(* Logix 5000 Rung export; software revision 16.04 *)

MODULES
   Local : vendor None type None code None
   MVI69E_AFC : vendor None type None code None
END_MODULES

TYPE AFCESiteAlarms :   // Indicates if a meter has any alarms
STRUCT
   Meter1 : BOOL;   // Meter in alarm
   Meter2 : BOOL;   // Meter in alarm
   Meter3 : BOOL;   // Meter in alarm
   Meter4 : BOOL;   // Meter in alarm
   Meter5 : BOOL;   // Meter in alarm
   Meter6 : BOOL;   // Meter in alarm
   Meter7 : BOOL;   // Meter in alarm
   Meter8 : BOOL;   // Meter in alarm
   Meter9 : BOOL;   // Meter in alarm
   Meter10 : BOOL;   // Meter in alarm
   Meter11 : BOOL;   // Meter in alarm
   Meter12 : BOOL;   // Meter in alarm
   Meter13 : BOOL;   // Meter in alarm
   Meter14 : BOOL;   // Meter in alarm
   Meter15 : BOOL;   // Meter in alarm
   Meter16 : BOOL;   // Meter in alarm
END_STRUCT
END_TYPE

TYPE AFCEMeterDifferentialLiquidArchive :   // Different Liquid Archive
STRUCT
   Write : AFCEMeterDifferentialLiquidArchiveWrite;
   Fetch : AFCEMeterDifferentialLiquidArchiveFetch;
END_STRUCT
END_TYPE

TYPE AFCEMeterDifferentialLiqCalRequest :
STRUCT
   ProcessVariable : AFCEMeterDifferentialLiqCalRequestProces;   // Process Variable
   ActionType : AFCEMeterCalRequestActionType;   // Action Type
   Value : AFCEMeterCalRequestActionValue;   // Value
   Count : DINT;   // Number of calibration requests
END_STRUCT
END_TYPE

TYPE AFCEFlag :   // Flags contains status information updated by ladder and also trigger bits for clock update
STRUCT
   AFCStopped : BOOL;   // Indicates that the module has sent a new input block to be processed by ladder - UPDATED BY LADDER
   AFCInputSequenceNum : INT;   // Meter number (0 -15) associated to blocks 1-16. Used to update "Profile" (meter type and product group.) UPDATED BY LADDER
END_STRUCT
END_TYPE

TYPE AFCEUtilBlockNonInterrupt :
STRUCT
   Now : BOOL;
   ModbusMasterCommand : BOOL;
   ModbusMasterResponse : BOOL;
   Archive : DINT;
   Prover : BOOL;
   PassThru : BOOL;
   Calibration : BOOL;
END_STRUCT
END_TYPE

TYPE AFCEMeterCalRequestActionType :
STRUCT
   ZeroShift : BOOL;   // Zero Shift
   SetZero : BOOL;   // Set Zero
   SetSpan : BOOL;   // Set Span
   SetMid1 : BOOL;   // Set Mid 1
   SetMid2 : BOOL;   // Set Mid 2
   SetMid3 : BOOL;   // Set Mid 3
END_STRUCT
END_TYPE

TYPE AFCEMeterDifferentialLiqCal :   // Processor Mediated Calibration
STRUCT
   Request : AFCEMeterDifferentialLiqCalRequest;   // Calibration Request from module
   Response : AFCEMeterCalResponse;   // Processor Response
END_STRUCT
END_TYPE

TYPE AFCEProveConfigEnable :   // Prove controls at enable
STRUCT
   MeterNumber : INT;   // Meter number requested (1-16)
   AutoAcceptProve : BOOL;   // Auto-accept the prove
   AutoContinueProve : BOOL;   // Auto-continue the prove
END_STRUCT
END_TYPE

TYPE AFCEModbusGateway :   // Modbus Gateway
STRUCT
   Command : AFCEModbusGatewayCommand[10];   // Modbus gateway commands - contains setup and modbus data
END_STRUCT
END_TYPE

TYPE AFCEMeterCalRequestActionValue :
STRUCT
   ZeroShift : AFCEMeterCalRequestValue;   // Zero Shift
   SetZero : AFCEMeterCalRequestValue;   // Set Zero
   SetSpan : AFCEMeterCalRequestValue;   // Set Span
   SetMid1 : AFCEMeterCalRequestValue;   // Set Mid 1
   SetMid2 : AFCEMeterCalRequestValue;   // Set Mid 2
   SetMid3 : AFCEMeterCalRequestValue;   // Set Mid 3
END_STRUCT
END_TYPE

TYPE AFCEMeterDifferentialLiquidArchiveWrite :   // Write Archive
STRUCT
   Daily : BOOL;   // Set to 1 to write daily archive
   Hourly : BOOL;   // Set to 1 to write hourly archive
END_STRUCT
END_TYPE

TYPE AFCEMeterAnalysisError :
STRUCT
   StreamOutOfRange : BOOL;   // Requested Stream Number Out of Range
   StreamNotConfigured : BOOL;   // Requested Stream Not Configured
END_STRUCT
END_TYPE

TYPE AFCEMeterCalRequestValue :
STRUCT
   Applied : REAL;   // Applied
   Measured : REAL;   // Measured
END_STRUCT
END_TYPE

TYPE AFCEModbusMasterDataType :   // Modbus master data type
STRUCT
   Bit : BOOL;   // bit type
   Word : BOOL;   // word type (16-bit)
   Long : BOOL;   // long integer (32-bit)
   LongRemote : BOOL;   // long integer (32-bit)
END_STRUCT
END_TYPE

TYPE AFCEUtil :   // Used for internal ladder logic usage. These values must not be changed by user application.
STRUCT
   Flags : AFCEFlag;   // Wallclock update commands
   CycleCounter : INT;   // Reflects current block ID calculated by ladder to be sent to the module
   Buffer : AFCEUtilBuffer;
   Block : AFCEUtilBlock;
END_STRUCT
END_TYPE

TYPE AFCEWallclock :
STRUCT
   GetAFCTime : BOOL;   // Get current AFC Time
   SetAFCTimeFromPLCTime : BOOL;   // Set AFC time from PLC time. Updates current AFC time
   EnableLocalDateTime : BOOL;   // Enable Local Date Time.
   AFCTime : AFCETime;   // Coordinated Universal Time. Updated by either getting or setting AFC time.
END_STRUCT
END_TYPE

TYPE AFCEMeterDifferentialLiquidAlarmControl :   // Differential Liquid Process Alarms
STRUCT
   DifferentialPressure : AFCEMeterProcessAlarm;   // Differential Pressure Alarms
   FlowRate : AFCEMeterProcessAlarm;   // Flow Rate
   Temperature : AFCEMeterProcessAlarm;   // Temperature Alarms
   Pressure : AFCEMeterProcessAlarm;   // Pressure Alarms
   Density : AFCEMeterProcessAlarm;   // Density Alarms
   WaterPercent : AFCEMeterProcessAlarm;   // Differential Pressure Alarms
END_STRUCT
END_TYPE

TYPE AFCEProvePhaseBitmap :   // AFC prove phase bitmap
STRUCT
   NotSelected : BOOL;   // Not selected
   Active : BOOL;   // Active, not counting
   CountingPast1stSwitch : BOOL;   // Counting past 1st switch for Udir and forward leg for Bdir)
   Past2ndSwitchFwdLeg : BOOL;   // Past 2nd switch forward leg (bidirectional only)
   Past1stSwithRetLeg : BOOL;   // Past 1st switch return leg (bidirectional only)
   RunComplete : BOOL;   // Run complete. past 2nd switch.
END_STRUCT
END_TYPE

TYPE AFCEProveInputConfig :   // Prove input block results - prover configuration
STRUCT
   Type : INT;   // Prover type
   Options : INT;   // Prover options
   RunsPerProveTotal : INT;   // Total runs per prove
   RunsPerProveSelected : INT;   // Selected runs per prove
   MaxRunsBeforeAbort : INT;   // Max total runs before abort
   ShortPassesPerRun : INT;   // Short passes per run if bidir = 2 , else 0
END_STRUCT
END_TYPE

TYPE AFCEMeterCalResponse :
STRUCT
   Trigger : BOOL;   // Send Error Code and Values to module to be recorded
   ErrorCode : SINT;   // Error Code to send. 0-4 allowed. 0=No error. 1-4=User defined.
   Value : AFCEMeterCalRequestValue;   // Value to Send
   Count : DINT;   // Number of calibration responses
END_STRUCT
END_TYPE

TYPE AFCEMeterDifferentialLiqBackPlaneReturn :   // Differential Liquid Meter
STRUCT
   StandardDefault : AFCEMeterDifferentialLiqStandardDataDflt;
   StandardRaw : INT[14];
   Extended : AFCEExtended;
END_STRUCT
END_TYPE

TYPE AFCEMeterDifferentialLiquidProcess :   // Differential Liquid Process Variables
STRUCT
   DifferentialPressure : REAL;   // Differential pressure if Primary Input = Differential pressure
   FlowRate : REAL;   // Flow Rate if Primary Input = Flow Rate
   Temperature : REAL;   // Temperature
   Pressure : REAL;   // Static Pressure
   Density : REAL;   // Density
   WaterPercent : REAL;   // Water %
END_STRUCT
END_TYPE

TYPE AFCEMeterArchiveFetchError :
STRUCT
   ArchiveSelectionInvalid : BOOL;   // Archive File Selection Invalid
   AgeOutsideSize : BOOL;   // Age Outside Configured File Size
   ArchiveNeverWritten : BOOL;   // Age OK but Archive Record Never Written (new or reconfigured meter)
   Reserverd1 : BOOL;
   Reserverd2 : BOOL;
   Reserverd3 : BOOL;
   Reserverd4 : BOOL;
   Reserverd5 : BOOL;
   Reserverd6 : BOOL;
   Reserverd7 : BOOL;
   Reserverd8 : BOOL;
   Reserverd9 : BOOL;
   Reserverd10 : BOOL;
   Reserverd11 : BOOL;
   Reserverd12 : BOOL;
   Reserverd13 : BOOL;
END_STRUCT
END_TYPE

TYPE AFCEModbusGatewayCommand :   // Modbus Gateway Command
STRUCT
   Config : AFCEModbusGatewayConfig;   // Config data to be entered by the user.
   Trigger : BOOL;   // Trigger the Command, when cleared module has responded.
   Data : INT[200];   // Contains modbus data written to the module (write commands)
END_STRUCT
END_TYPE

TYPE AFCEProveConfigAccept :   // Prove controls at accept. If auto-accept is selected must be available at enable
STRUCT
   RequestedInterpolationPoint : INT;   // Requested interpolation point (0 nearest)
   ApplyMFChangeAllStreams : BOOL;   // Apply change in meter factor to all streams
   ApplyMFChangeCurve : BOOL;   // Apply change in meter factor to all curve points
   ApplyNewMF : BOOL;   // CApply new meter factor
END_STRUCT
END_TYPE

TYPE AFCEModbusMasterCommand :   // Modbus Master Command
STRUCT
   Config : AFCEModbusMasterConfig;   // Modbus Master Configuration
   ErrorCode : INT;   // Error Code associated to Modbus Master Command
   Pending : BOOL;   // Pending Modbus Master Command - waiting for Modbus Response
   ReturnedTransactionID : DINT;   // Changes to Config.TransactionID value when response has returned.
   Data : INT[100];   // Read or Write Data
END_STRUCT
END_TYPE

TYPE AFCEMeterStatusMeter :   // Meter Status
STRUCT
   Enabled : BOOL;   // Meter Enable Status, 1=enabled
   EnableAlarm : BOOL;   // If set either: 1. The meter is not configured. 2. The event log is full, the action was not performed.
END_STRUCT
END_TYPE

TYPE AFCEMeterControl :   // Enable/Disable Meter and Streams
STRUCT
   Meter : AFCEMeterControlMeter;   // Control the Meter
   Stream : AFCEMeterControlStream;   // Control the Meter Streams
   ResetAccumulators : AFCEMeterSignals;   // Resets for meter accumulators
END_STRUCT
END_TYPE

TYPE AFCEProveSequencing :   // AFC prove sequencing tag for phase selection and ball positioning
STRUCT
   Phase : AFCEProvePhaseBitmap;   // AFC phase sequencing
   BallPositionReady : BOOL;   // Ball position: Ready (Udir & Bdir only; fwd leg Bdir)
   BallPositionSealed : BOOL;   // Ball position: Sealed (Udir & Bdir only; fwd leg Bdir)
   BallPositionReadyBwdLeg : BOOL;   // Ball position: Ready bwd leg (Bdir only)
   BallPositionSealedBwdLeg : BOOL;   // Ball position: Sealed bwd leg (Bdir only)
END_STRUCT
END_TYPE

TYPE AFCEMeterDifferentialLiquidAlarm :
STRUCT
   Control : AFCEMeterDifferentialLiquidAlarmControl;   // Alarm Control
END_STRUCT
END_TYPE

TYPE AFCEUtilBlockInterrupt :
STRUCT
   Now : BOOL;
   ModbusGateway : DINT;
   EnableDisable : BOOL;
   Analysis : DINT;
END_STRUCT
END_TYPE

TYPE AFCEMeterDifferentialLiqStandardDataDflt :   // EAFC Backplane Return Standard Data
STRUCT
   Meter_Alarms : DINT;   // Meter alarms
   NR_Acc_Net_Totalizer : DINT;   // Non-resettable accumulator, net, totalizer (m3)
   NR_Acc_Net_Residue : REAL;   // Non-resettable accumulator, net, residue (m3)
   FlowRate_Net : REAL;   // Flow rate, net (m3/h)
   NR_Acc_Gross_Totalizer : DINT;   // Non-resettable accumulator, gross, totalizer (m3)
   NR_Acc_GrossStandard_Totalizer : DINT;   // Non-resettable accumulator, gross standard, totalizer (m3)
   NR_Acc_Mass_Totalizer : DINT;   // Non-resettable accumulator, mass, totalizer (kg)
END_STRUCT
END_TYPE

TYPE AFCEComponents :   // High precision gas component analysis (only supported version 2.07.000)
STRUCT
   C1 : REAL;   // Methane
   N2 : REAL;   // Nitrogen
   CO2 : REAL;   // Carbon Dioxide
   C2 : REAL;   // Ethane
   C3 : REAL;   // Propane
   H20 : REAL;   // Water
   H2S : REAL;   // Hydrogen Sulphide
   H2 : REAL;   // Hydrogen
   CO : REAL;   // Carbon Monoxide
   O2 : REAL;   // Oxygen
   IC4 : REAL;   // Iso-butane
   NC4 : REAL;   // Normal Butane
   IC5 : REAL;   // Iso-pentane
   NC5 : REAL;   // Normal-pentane
   C6 : REAL;   // Hexane
   C7 : REAL;   // Heptane
   C8 : REAL;   // Octane
   C9 : REAL;   // Nonane
   C10 : REAL;   // Decane
   He : REAL;   // Helium
   Ar : REAL;   // Argon
   NeoC5 : REAL;   // Not Used
   UxUser1 : REAL;   // Not Used
   UyUser2 : REAL;   // Not Used
   UxUser3 : REAL;   // Not Used
   UyUser4 : REAL;   // Not Used
   UxUser5 : REAL;   // Not Used
   UyUser6 : REAL;   // Not Used
   UxUser7 : REAL;   // Not Used
   UyUser8 : REAL;   // Not Used
   UxUser9 : REAL;   // Not Used
   UyUser10 : REAL;   // Not Used
END_STRUCT
END_TYPE

TYPE AFCEMeterStatus :   // Status
STRUCT
   Meter : AFCEMeterStatusMeter;   // Meter Status
   Stream : AFCEMeterStatusStream;   // Stream Status
END_STRUCT
END_TYPE

TYPE AFCEUtilBlock :
STRUCT
   ProcessInput : INT;
   InterruptPending : AFCEUtilBlockInterrupt;
   InterruptComplete : AFCEUtilBlockInterrupt;
   NonInterruptPending : AFCEUtilBlockNonInterrupt;
   NonInterruptComplete : AFCEUtilBlockNonInterrupt;
END_STRUCT
END_TYPE

TYPE AFCEModbusGatewayConfig :   // Modbus Ggateway Configuration
STRUCT
   Enable : BOOL;   // Set to 1 to enable modbus gateway command (0=disable)
   StartRegister : DINT;   // Start modbus address
   RegisterCount : INT;   // Word count (200 max)
   FunctionType : BOOL;   // 0 = read command, 1 = write command
   RegisterType : BOOL;   // 0 = holding register, 1 = input register
   SlaveType : BOOL;   // 0 = primary slave, 1 = virtual slave
END_STRUCT
END_TYPE

TYPE AFCEMeterControlMeter :   // Enable and Disable Meter
STRUCT
   Enable : BOOL;   // Enable the Meter
   Disable : BOOL;   // Disable the Meter
END_STRUCT
END_TYPE

TYPE AFCEMeterProfile :   // Meter configuration profile
STRUCT
   MeterType : BOOL;   // 0=Differential, 1=Linear
   ProductGroup : BOOL;   // 0=Gas, 1=Liquid
   PrimaryInput : BOOL;   // For differential, 0=Differential Pressure 1=Flow Rate. For Linear, 0=Pulse Count 1=Pulse Frequency
   AOIMismatch : BOOL;   // AOI Meter type does not match module for meter number
END_STRUCT
END_TYPE

TYPE AFCEModbusPassThru :   // AFC Modbus Pass-thru
STRUCT
   Enable : BOOL;   // Set to 1 to enable pass-thru functionality (requires AFC Manager setting)
   MessagePresent : BOOL;   // Message present in the response block
   GetMessage : BOOL;   // Get the pass-thru message. When the bit is cleared the message has been transferred to the PLC.
   FunctionBitWrite : BOOL;   // Function bit write
   OverflowError : BOOL;   // Overflow error flag
   ModbusAddress : INT;   // Destination modbus address
   RegisterCount : INT;   // Number of elements associated to command
   ReadDataWord : INT[125];   // Contains received data for word commands
   ReadDataBit : AFCEModbusPassThruBitData;   // Contains received data for bit commands
END_STRUCT
END_TYPE

TYPE AFCEUtilBuffer :   // Buffer
STRUCT
   Input : INT[248];   // Input buffer contains the complete block to be copied from the module
   Output : INT[247];   // Output buffer contains data the complete block to be copied to the module
   Process : INT[180];
   ArchiveDay : INT[98];
   ArchiveHour : INT[98];
   Prove : INT[26];
   Analysis : INT[198];
   MeterEnableDisable : INT[4];
   StreamEnable : INT[36];
   StreamDisable : INT[36];
   StreamSelect : INT[24];
   MeterSignals : INT[24];
   Calibration : INT[36];
END_STRUCT
END_TYPE

TYPE AFCEProveStatus :   // Status of the prove (returned from the module to the processor)
STRUCT
   ProveAccepted : BOOL;   // Prove was accepted
   MeterFactorApplied : BOOL;   // Meter factor was applied
   MFAppliedToCurve : BOOL;   // Meter factor was applied to all points in the curve
   MFAppliedToStreams : BOOL;   // Meter factor was applied to all streams
   ProveRejectedByCommand : BOOL;   // Prove was rejected by command
   ProveRejectedNoRuns : BOOL;   // Prove was rejected - empty prove (no runs)
   ProveRejectedDivideBy0 : BOOL;   // Prove was rejected - divide by 0
   ProveEnabled : BOOL;   // Prove is enabled
   ProvingRunInProgress : BOOL;   // Proving run is in progress
   ProveRejectedAbort : BOOL;   // Prove rejected: abort
   ProvePaused : BOOL;   // Prove is paused
   RunCancelled : BOOL;   // Run Is cancelled
   RunTimedOut : BOOL;   // Run timed out
END_STRUCT
END_TYPE

TYPE AFCEMeterStatusStreamAlarm :   // Stream Alarms
STRUCT
   StreamOutOfRange : BOOL;   // Requested Stream Number Out of Range
   StreamNotConfigured : BOOL;   // Requested Stream not Configured
   StreamNotEnabled : BOOL;   // Requested Stream not Enabled
   EventLogFull : BOOL;   // Event Log Full, Action not Performed
END_STRUCT
END_TYPE

TYPE AFCEMeterDifferentialLiquidArchiveFetch :
STRUCT
   Daily : AFCEMeterDifferentialLiquidArchiveFetchT;
   Hourly : AFCEMeterDifferentialLiquidArchiveFetchT;
END_STRUCT
END_TYPE

TYPE AFCEProveConfig :   // Controls (configuration settings) associated to the prover
STRUCT
   Enable : AFCEProveConfigEnable;   // Controls at enable
   Accept : AFCEProveConfigAccept;   // Controls at accept
END_STRUCT
END_TYPE

TYPE AFCESiteStatus :   // Site status bits - contains general information about the module - not meter specific
STRUCT
   AFCActive : BOOL;   // AFC active
   ChecksumAlarms : BOOL;   // Checkum alarm active
   Reserved2 : BOOL;
   Reserved3 : BOOL;
   PLCHalted : BOOL;   // PLC in program mode or missing
   CfgChanged : BOOL;   // Configuration changed
   Powerup : BOOL;   // Module powered up
   ColdStart : BOOL;   // Module performed cold start (BBRAM initialized)
   ModbusMasterPending : BOOL;   // Modbus Master Poll Pending
   ModbusMasterComplete : BOOL;   // Modbus Master Poll Complete
   ModbusPassThruPending : BOOL;   // Modbus Pass-thru Input Pending
   CalibrationRequest : BOOL;   // Calibration request from module
   ProverEnabled : BOOL;   // Prover Enabled
   Reserved13 : BOOL;
   Reserved14 : BOOL;
   Reserved15 : BOOL;
END_STRUCT
END_TYPE

TYPE AFCEModbusMaster :   // Modbus Master. Port 3 must be configured as modbus master through AFC Manager to use this feature.
STRUCT
   Enable : BOOL;   // Enable the modbus master funcionality
   CommandIndex : INT;   // Selects which command index will be executed
   Command : AFCEModbusMasterCommand[10];   // Each command contains a specific modbus request to be sent out of the port
END_STRUCT
END_TYPE

TYPE AFCEProveProcess :   // Prove process output from processor to the module
STRUCT
   Sequencing : AFCEProveSequencing;   // Prover sequencing
   Temperature : REAL;   // Temperature for Single Probe provers. And Inlet Temperature for Dual Probe Provers.
   OutletTemperature : REAL;   // Outlet Temperature for Provers with Dual Probes.
   SwitchBarTemperature : REAL;   // Switch bar temperature
   Pressure : REAL;   // Pressure for Single Probe provers. And Inlet Pressure for Dual Probe Provers.
   OutletPressure : REAL;   // Outlet Pressure for Provers with Dual Probes.
   ProverDensity : REAL;   // Prover density
END_STRUCT
END_TYPE

TYPE AFCEExtended :
STRUCT
   Trigger : BOOL;
   Data : AFCEExtendedData;
END_STRUCT
END_TYPE

TYPE AFCEMeterSignals :   // Meter trigger accumulator and archive resets
STRUCT
   ResetAccumulator1 : BOOL;   // Set to 1 to reset resettable accumulator 1
   ResetAccumulator2 : BOOL;   // Set to 1 to reset resettable accumulator 2
   ResetAccumulator3 : BOOL;   // Set to 1 to reset resettable accumulator 3
   ResetAccumulator4 : BOOL;   // Set to 1 to reset resettable accumulator 4
END_STRUCT
END_TYPE

TYPE AFCEMeterProcessAlarm :   // Process Alarms
STRUCT
   SetGeneralFail : BOOL;   // Set to indicate General Failure of the Transmitter
   StaleData : BOOL;   // Clear to Indicate new process input data
   SetLowThreshold : BOOL;   // Set to indicate Lower Range Limit Exceeded
   SetHighThreshold : BOOL;   // Set to indicate Upper Range Limit Exceeded
   SetAutoClearStaleData : BOOL;   // Set to automatically clear stale data
END_STRUCT
END_TYPE

TYPE AFCETime :   // AFC time format used for wallclock update.
STRUCT
   Year : DINT;   // Year
   Month : DINT;   // Month
   Day : DINT;   // Day
   Hour : DINT;   // Hour
   Minute : DINT;   // Minute
   second : DINT;   // Seconds
END_STRUCT
END_TYPE

TYPE AFCEModbusMasterSwap :   // Modbus master swap words/ swap bytes
STRUCT
   SwapWords : BOOL;   // Swap words
   SwapBytes : BOOL;   // Swap bytes
END_STRUCT
END_TYPE

TYPE AFCEMeterControlStream :
STRUCT
   Selected : SINT;   // Stream to Enable or Disable and/or make active.
   EnableSelected : BOOL;   // Enable the Selected Stream
   DisableSelected : BOOL;   // Disable the Selected Stream
   SetSelectedToActive : BOOL;   // Set Selected to Active Stream
END_STRUCT
END_TYPE

TYPE AFCEMeterDifferentialLiqCalRequestProces :
STRUCT
   DifferentialPressure : BOOL;   // Differential Pressure
   Temperature : BOOL;   // Temperature
   Pressure : BOOL;   // Pressure
   Density : BOOL;   // Density
   WaterContent : BOOL;   // Water Content
END_STRUCT
END_TYPE

TYPE AFCEMeterDifferentialLiquid :   // Differential Liquid Meter
STRUCT
   Control : AFCEMeterControl;   // Meter Control
   Status : AFCEMeterStatus;   // Meter Status
   ProcessVariables : AFCEMeterDifferentialLiquidProcess;   // Input process variables to be transferred to the module
   Analysis : AFCEMeterAnalysis;   // Molar Analysis data to be transferred to the module (only for gas products with online gas chromatograph applications)
   Alarm : AFCEMeterDifferentialLiquidAlarm;   // Meter Alarms
   Archive : AFCEMeterDifferentialLiquidArchive;   // Archive
   Profile : AFCEMeterProfile;   // Module profile (meter type/product group) transfered from the module
   Calibration : AFCEMeterDifferentialLiqCal;   // Calibration
   BackPlaneReturn : AFCEMeterDifferentialLiqBackPlaneReturn;
END_STRUCT
END_TYPE

TYPE AFCEProvePulseCount :   // Values to be supplied at the end of the pass/run
STRUCT
   Meter : DINT;   // Meter pulse count
   MasterMeter : DINT;   // Master meter pulse count
END_STRUCT
END_TYPE

TYPE AFCEMeterStatusStream :
STRUCT
   Active : INT;   // Current Active Stream
   Enabled : AFCEMeterStatusStreamEnabled;   // Enabled Streams
   Configured : AFCEMeterStatusStreamEnabled;   // Configured Streams
   EnableAlarm : AFCEMeterStatusStreamAlarm;   // Enable Alarms
END_STRUCT
END_TYPE

TYPE AFCEExtendedData :
STRUCT
   Raw : INT[64];
END_STRUCT
END_TYPE

TYPE AFCEModbusPassThruBitData :   // AFC Modbus Pass-thru Bit Data
STRUCT
   Data : BOOL[2016];   // Contains received data for bit commands
END_STRUCT
END_TYPE

TYPE AFCEMeterDifferentialLiquidArchiveDflt :   // Default Configuration
STRUCT
   ClosingTimestamp : DINT;
   CumulativeActiveStreams : INT;
   CurrentActiveStream : SINT;
   MeterStatus : SINT;
   FlowingPeriod : DINT;
   PeriodDuration : DINT;
   AccumulatorTotalizer : DINT;
   AccumulatorResidue : REAL;
   MeterAlarms : DINT;
   PrimaryInput : REAL;   // Either Differential Pressure or Flow Rate
   Temperature : REAL;
   Pressure : REAL;
   Density : REAL;
   WaterContent : REAL;
   ReferenceDensity : REAL;
   Ctpl : REAL;
   AGA3DensityExtension : REAL;
   AGA3CoefficientDischarge : REAL;
   Available01 : INT;
   Available02 : INT;
   Cprime : REAL;
   MassNRAccumulatorCurrent : REAL;   // Non-resettable
   MassNRAccumulatorOpening : REAL;   // Non-resettable
   Available03 : INT;
   Available04 : INT;
   Available05 : INT;
   Available06 : INT;
   NetNRAccumulatorCurrent : REAL;   // Non-resettable
   NetNRAccumulatorOpening : REAL;   // Non-resettable
   GrossNRAccumulatorCurrent : REAL;   // Non-resettable
   GrossNRAccumulatorOpening : REAL;   // Non-resettable
   GrossStandardNRAccumulatorOpening : REAL;   // Non-resettable
   GrossStandardNRAccumulatorCurrent : REAL;   // Non-resettable
   WaterNRAccumulatorCurrent : REAL;   // Non-resettable
   WaterNRAccumulatorOpening : REAL;   // Non-resettable
   API2540VaporPressureAbs : REAL;   // Non-resettable
   Available07 : INT;
   Available08 : INT;
   UserSpecifiedFlowAverage1 : REAL;
   UserSpecifiedFlowAverage2 : REAL;
   UserSpecifiedFlowAverage3 : REAL;
END_STRUCT
END_TYPE

TYPE AFCEModbusMasterConfig :   // Modbus master command settings
STRUCT
   Enable : BOOL;   // Set to 1 to enable command (0=disable)
   FunctionType : BOOL;   // Set to 1 to select write command (0=read command)
   RegisterBank : BOOL;   // Set to 1 to select input register (0=holding register)
   DataType : AFCEModbusMasterDataType;   // Select data type format
   SwapOption : AFCEModbusMasterSwap;   // Select byte and word swap (1 = swap, 0 = no swap)
   TypeSwap : INT;   // This value is calculated by ladder logic and must not be modified by user
   SlaveAddress : INT;   // Modbus slave address of remote device
   ModbusAddress : INT;   // Modbus data address on remote slave
   ElementCount : INT;   // Number of data elements (125 words)
   TransactionID : INT;   // Transaction ID. This value is returned to the ReturnedTransaction ID when the response has been received.
END_STRUCT
END_TYPE

TYPE AFCEMeterDifferentialLiquidArchiveFetchT :   // Fetch Archive
STRUCT
   Trigger : BOOL;   // Trigger Archive Fetch
   Age : INT;   // 0 = Current Archive
   Error : AFCEMeterArchiveFetchError;   // Archive Fetch Error
   Default : AFCEMeterDifferentialLiquidArchiveDflt;   // Default Archive
   Raw : INT[100];   // Raw Archive
END_STRUCT
END_TYPE

TYPE AFCEModuleDef :   // Main user defined data type
STRUCT
   ModbusGateway : AFCEModbusGateway;   // Reads and write data between processor and module modbus table
   ModbusMaster : AFCEModbusMaster;   // Setup modbus master commands to be sent to remote slaves (through Port 3)
   ModbusPassThru : AFCEModbusPassThru;   // Modbus pass-thru data
   SiteStatus : AFCESiteStatus;   // Site status
   MeterAlarms : AFCESiteAlarms;   // Meter Alarms
   Prove : AFCEProve;   // Prover
   Wallclock : AFCEWallclock;   // Set clock and get clock information
   Firmware : AFCEFirmwareVersion;   // Firmware information
   Util : AFCEUtil;   // Used by ladder logic
END_STRUCT
END_TYPE

TYPE AFCEMeterAnalysis :   // Meter analysis components. Allows the processor to update molar analysis for low precision and high precision streams.
STRUCT
   Trigger : BOOL;   // Set to 1 to Send Updated Component Data to the Module
   Stream : INT;   // Stream for Analysis. Select 0 for current active stream.
   Error : AFCEMeterAnalysisError;   // Analysis Error
   Components : AFCEComponents;   // High precision gas components (floating point per component). Only supported for firmware version 2.07.000 or later
END_STRUCT
END_TYPE

TYPE AFCEProveSignals :   // Contains the proving signals that will trigger specific tasks from the module
STRUCT
   EnableProve : BOOL;   // Enables the prove
   AcceptProve : BOOL;   // Accepts the prove
   RejectProve : BOOL;   // Reject the prove
   RunStart : BOOL;   // Starts the run
   RunComplete : BOOL;   // Flags that the run is complete
   RunCancel : BOOL;   // Cancels the run
   RunDelete : BOOL;   // Deletes the run
   PassComplete : BOOL;   // Flag that the pass is complete
   PauseProve : BOOL;   // Pauses the Proving Process
   AbortProve : BOOL;   // Aborts the prove
END_STRUCT
END_TYPE

TYPE AFCEFirmwareVersion :
STRUCT
   Major : SINT;   // Major Version number
   Minor : SINT;   // Minor Version number
   Revision : INT;   // Revision
END_STRUCT
END_TYPE

TYPE AFCEProveRunResults :   // Run results of the prove. Copied from the module to the pocessor
STRUCT
   CountAttempted : INT;   // Run count attempted
   CountCompleted : INT;   // Run count completed
   CountSelected : INT;   // Run count selected
   RunsSelected : INT;   // Bit Mapped Runs selected for calculations from completed runs
   NewMeterFactor : REAL;   // New meter factor
   ChangeInMeterFactor : REAL;   // Change in meter factor
END_STRUCT
END_TYPE

TYPE AFCEMeterStatusStreamEnabled :   // Stream Status 1 = Enabled
STRUCT
   Stream1 : BOOL;
   Stream2 : BOOL;
   Stream3 : BOOL;
   Stream4 : BOOL;
   Stream5 : BOOL;
   Stream6 : BOOL;
   Stream7 : BOOL;
   Stream8 : BOOL;
   Stream9 : BOOL;
   Stream10 : BOOL;
   Stream11 : BOOL;
   Stream12 : BOOL;
   Stream13 : BOOL;
   Stream14 : BOOL;
   Stream15 : BOOL;
   Stream16 : BOOL;
END_STRUCT
END_TYPE

TYPE AFCEProve :   // Prove
STRUCT
   Process : AFCEProveProcess;   // Process Variables
   Signals : AFCEProveSignals;   // AFC Prove Signals (triggers the proving update)
   Config : AFCEProveConfig;   // AFC Prove Control (configuration settings)
   PulseCounts : AFCEProvePulseCount;   // Pulse counts to be updated at the end of the run/pass
   ConfigInput : AFCEProveInputConfig;   // AFC prover input configuration
   Status : AFCEProveStatus;   // AFC prover status
   ErrorCode : INT;   // Prove error code
   ProveControlsEcho : INT;   // AFC module Echos the state of the Prove Controls
   RequestedMeterEcho : INT;   // AFC module Echos the Meter number requested
   RequestedCurvePointEcho : INT;   // AFC module Echos the requested Curve Point
   RunResults : AFCEProveRunResults;   // Prove and run results
   ProveEnabled : BOOL;   // ON if prove is enabled. This flag is coped from inputbuffer[247]
END_STRUCT
END_TYPE

ADD_ON_INSTRUCTION AOI69EAFCMeterDifferentialLiquid   (* revision 1.6, vendor ProSoft Technology Inc., ExecutePrescan *)
// Add-On instruction for the MVI69E-AFC.
// Differential Liquid Meter
// Revision note:
// Updated  BackplaneReturn Tag name from ProcessInputs to Standard
// and ComponentAnalysis to Extended
// Help:
// v1.1:Compatible with version 4.04 of MVI69E-AFC firmware or higher.
// v1.1: Comp Analysis Return fix
// v1.2: Added Flow Rate Process Input and Flow Rate Alarm Controller Tags for Flow Rate Devices (and not just for Differential Pressure)
// v1.3: Addition of default process input backplane return data mapping.
// v1.4: Changed Prescan FLL instruction length from 240 words to 180 for proccess inputs. This stopped mismatch issue
// v1.4: Made correlation changes between the Module Archive Default UDTs and the AOI Archive Default UDTs.
// v1.5: Made changes to the Flow Rate Primary Input Block ID Insertion in Rung 8 (Removed +1),
// Modified ModbusGatewayConfig UDT StartRegister Tag Data Type from INT to DINT.
// v1.6: Updated Tags names AFCMeterXXYYYYYY.BackPlaneReturn.ProcessInputs to
// AFCMeterXXYYYYYY.BackPlaneReturn.Standard and
// AFCMeterXXYYYYYY.BackPlaneReturn.ComponentAnalysis
//  to AFCMeterXXYYYYYY.BackPlaneReturn.Extended.
VAR_IN_OUT
   ConnectionInput : INT[248]; {required}
   AFC : AFCEModuleDef; {required}
   AFCMeter : AFCEMeterDifferentialLiquid; {required}
END_VAR
VAR_INPUT
   MeterNumber : SINT; {required}   // Meter Number Set to a number between 1 and 16
END_VAR
VAR
   StreamSelectedShift : DINT;
   StreamSelectBuffer : INT;
   EnabledStatusBuffer : INT;
   StreamSelectBlockID : DINT;
   StreamNumberShift : DINT;
   StreamErrorBuffer : DINT;
   StreamEnableBlockID : DINT;
   StreamEnableBitPosition : DINT;
   StreamDisableBlockID : DINT;
   ProfileBuffer : SINT[2];
   ProcessInputBlockID : DINT;
   CalibrationHandleBuffer : INT;
   AnalysisGroupBitPosition : INT;
   ProcessAlarmShifter : DINT;
   ProcessAlarmHolder : DINT;
   ProcessAlarmBuffer : DINT;
   MeterSignaltBlockID : DINT;
   MeterNumberShift : DINT;
   MeterNumberBitPostition : DINT;
   Inputbuffer : INT[248];
   CalibrationMeterNumberBuffer : DINT;
   CalibrationMediationPending : BOOL;
   CalibrationInputScalingIndex : DINT;
   AnalysisErrorBuffer : INT;
   ArchiveStream : DINT;
   ArchiveMeterStatusRaw : DINT;
   ArchiveMeterStatusActiveStream : DINT;
   ArchiveCompleteBitCheck : DINT;
   ArchiveBlockID : DINT;
   AnalysisGroupShift : DINT;
   AnalysisCompleteBitCheck : DINT;
   AnalysisBufferOffset : DINT;
   AFCStopped : BOOL;
   AFCInputDataAvailable : BOOL;
   AnalysisBlockID : DINT;
END_VAR

ROUTINE Logic   (* ladder *)
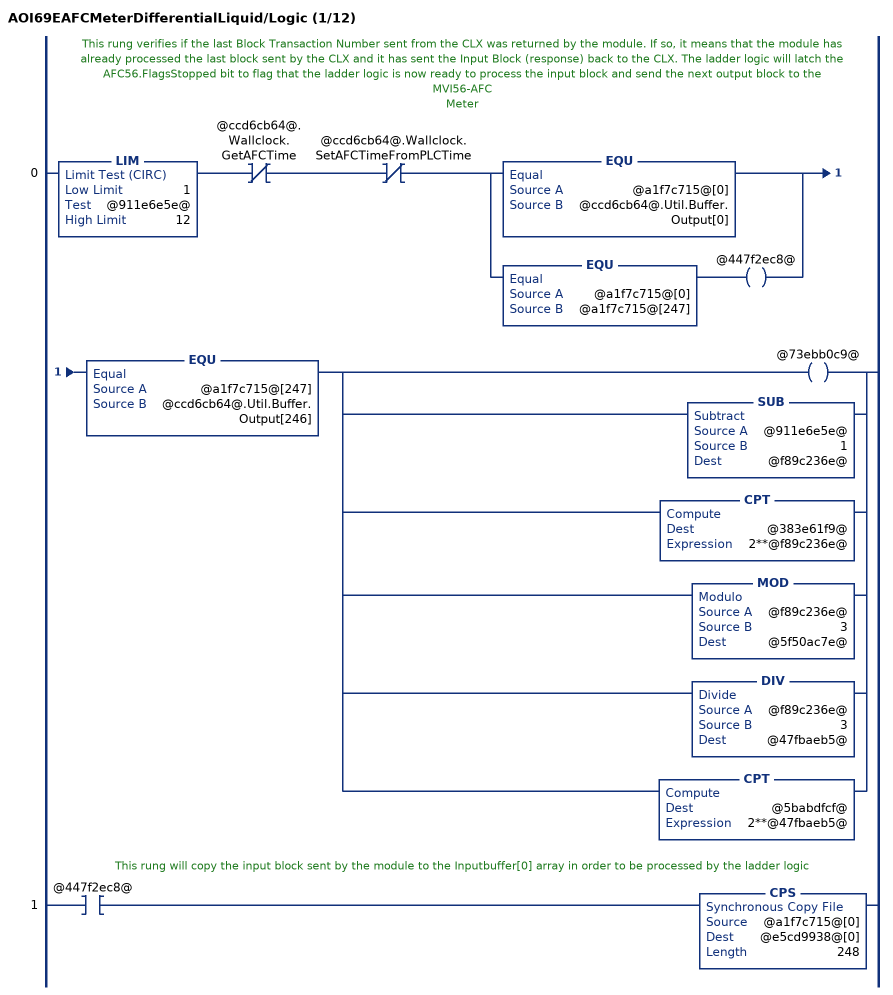
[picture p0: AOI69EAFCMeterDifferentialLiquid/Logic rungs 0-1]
   // This rung verifies if the last Block Transaction Number sent from the CLX was returned by the module. If so, it means that the module has already processed the last block sent by the CLX and it has sent the Input Block (response) back to the CLX. The ladder logic will latch the AFC56.FlagsStopped bit to flag that the ladder logic is now ready to process the input block and send the next output block to the MVI56-AFC
   // Meter
   0: LIM(1,@911e6e5e@,12)XIO(@ccd6cb64@.Wallclock.GetAFCTime)XIO(@ccd6cb64@.Wallclock.SetAFCTimeFromPLCTime)[EQU(@a1f7c715@[0],@ccd6cb64@.Util.Buffer.Output[0]) ,EQU(@a1f7c715@[0],@a1f7c715@[247]) OTE(@447f2ec8@) ]EQU(@a1f7c715@[247],@ccd6cb64@.Util.Buffer.Output[246])[OTE(@73ebb0c9@) ,SUB(@911e6e5e@,1,@f89c236e@) ,CPT(@383e61f9@,2**@f89c236e@) ,MOD(@f89c236e@,3,@5f50ac7e@) ,DIV(@f89c236e@,3,@47fbaeb5@) ,CPT(@5babdfcf@,2**@47fbaeb5@) ];
   // This rung will copy the input block sent by the module to the Inputbuffer[0] array in order to be processed by the ladder logic
   1: XIC(@447f2ec8@)CPS(@a1f7c715@[0],@e5cd9938@[0],248);
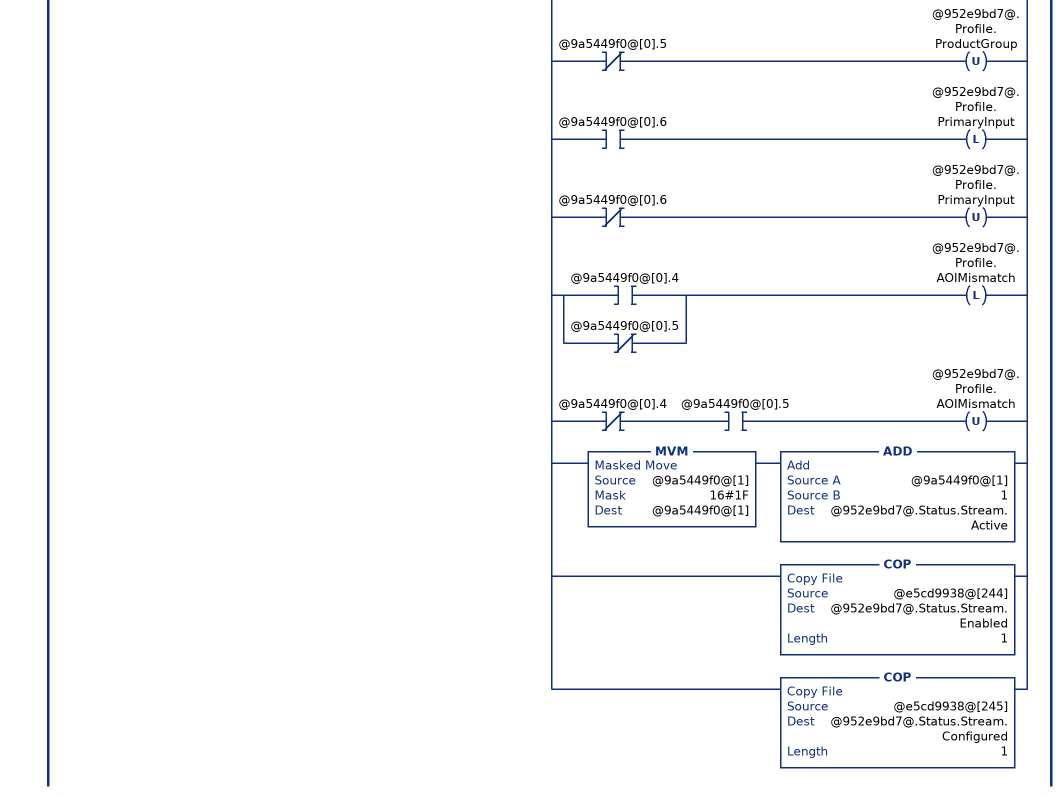
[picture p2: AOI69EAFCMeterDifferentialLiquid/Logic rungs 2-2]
   // Read process input backplane return and
   // meter profile (when block ID matches meter number).
   2: XIC(@447f2ec8@)LIM(1,@e5cd9938@[0],12)[COP(@e5cd9938@[3+@f89c236e@*15],@952e9bd7@.BackPlaneReturn.StandardRaw[0],14) ,COP(@952e9bd7@.BackPlaneReturn.StandardRaw[0],@952e9bd7@.BackPlaneReturn.StandardDefault,1) ,COP(@e5cd9938@[246],@ccd6cb64@.SiteStatus,1) ,EQU(@e5cd9938@[0],@911e6e5e@) [COP(@e5cd9938@[243],@9a5449f0@[0],2) ,[XIC(@9a5449f0@[0].0) OTL(@952e9bd7@.Status.Meter.EnableAlarm) ,XIO(@9a5449f0@[0].0) OTU(@952e9bd7@.Status.Meter.EnableAlarm) ] ,[XIC(@9a5449f0@[0].1) OTL(@952e9bd7@.Status.Meter.Enabled) ,XIO(@9a5449f0@[0].1) OTU(@952e9bd7@.Status.Meter.Enabled) ] ,[[XIC(@9a5449f0@[0].4) OTL(@952e9bd7@.Profile.MeterType) ,XIO(@9a5449f0@[0].4) OTU(@952e9bd7@.Profile.MeterType) ] ,[XIC(@9a5449f0@[0].5) OTL(@952e9bd7@.Profile.ProductGroup) ,XIO(@9a5449f0@[0].5) OTU(@952e9bd7@.Profile.ProductGroup) ] ,[XIC(@9a5449f0@[0].6) OTL(@952e9bd7@.Profile.PrimaryInput) ,XIO(@9a5449f0@[0].6) OTU(@952e9bd7@.Profile.PrimaryInput) ] ] ,[[XIC(@9a5449f0@[0].4) ,XIO(@9a5449f0@[0].5) ] OTL(@952e9bd7@.Profile.AOIMismatch) ,XIO(@9a5449f0@[0].4) XIC(@9a5449f0@[0].5) OTU(@952e9bd7@.Profile.AOIMismatch) ] ,MVM(@9a5449f0@[1],16#1F,@9a5449f0@[1]) ADD(@9a5449f0@[1],1,@952e9bd7@.Status.Stream.Active) ,COP(@e5cd9938@[244],@952e9bd7@.Status.Stream.Enabled,1) ,COP(@e5cd9938@[245],@952e9bd7@.Status.Stream.Configured,1) ] ];
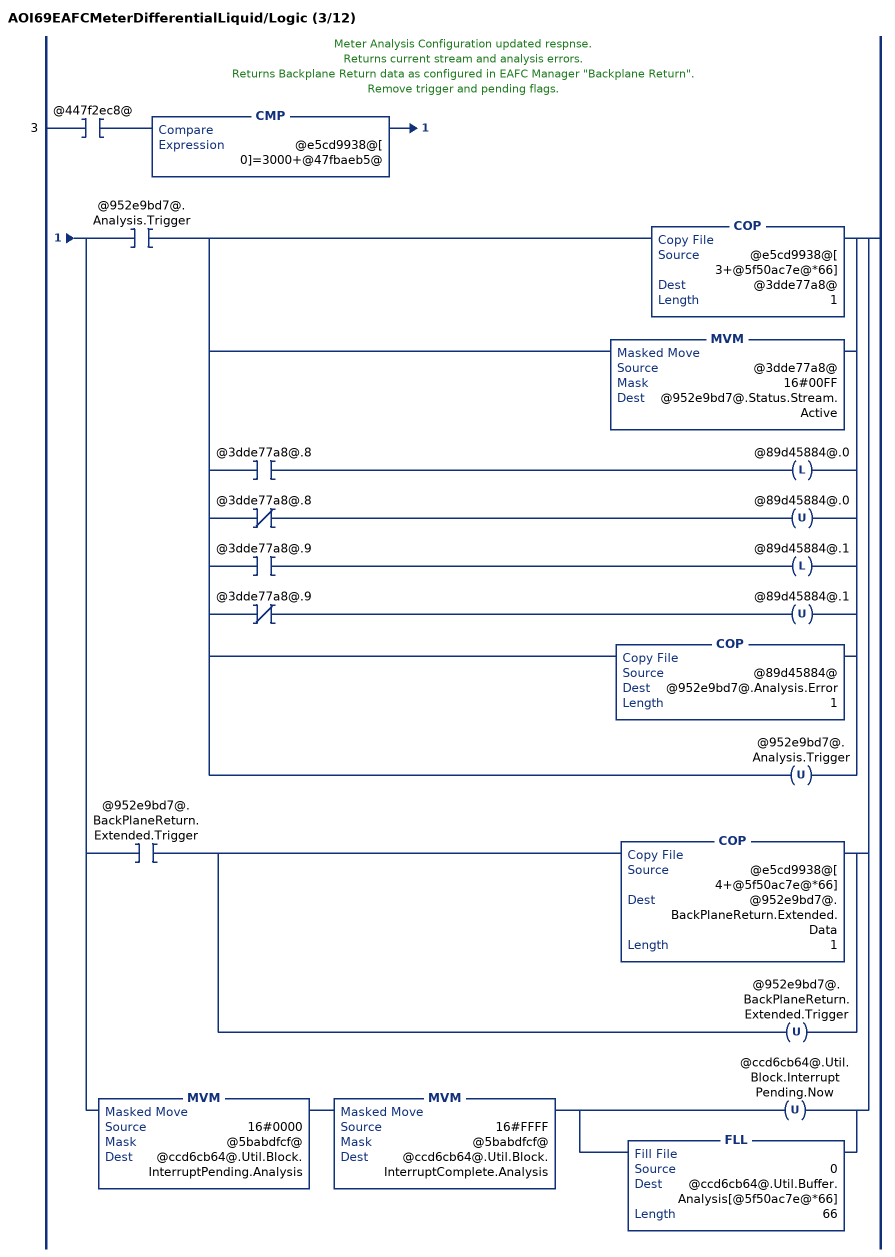
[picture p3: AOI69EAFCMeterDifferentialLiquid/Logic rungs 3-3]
   // Meter Analysis Configuration updated respnse.
   // Returns current stream and analysis errors.
   // Returns Backplane Return data as configured in EAFC Manager "Backplane Return".
   // Remove trigger and pending flags.
   3: XIC(@447f2ec8@)CMP(@e5cd9938@[0]=3000+@47fbaeb5@)[XIC(@952e9bd7@.Analysis.Trigger) [COP(@e5cd9938@[3+@5f50ac7e@*66],@3dde77a8@,1) ,MVM(@3dde77a8@,16#00FF,@952e9bd7@.Status.Stream.Active) ,[XIC(@3dde77a8@.8) OTL(@89d45884@.0) ,XIO(@3dde77a8@.8) OTU(@89d45884@.0) ] ,[XIC(@3dde77a8@.9) OTL(@89d45884@.1) ,XIO(@3dde77a8@.9) OTU(@89d45884@.1) ] ,COP(@89d45884@,@952e9bd7@.Analysis.Error,1) ,OTU(@952e9bd7@.Analysis.Trigger) ] ,XIC(@952e9bd7@.BackPlaneReturn.Extended.Trigger) [COP(@e5cd9938@[4+@5f50ac7e@*66],@952e9bd7@.BackPlaneReturn.Extended.Data,1) ,OTU(@952e9bd7@.BackPlaneReturn.Extended.Trigger) ] ,MVM(16#0000,@5babdfcf@,@ccd6cb64@.Util.Block.InterruptPending.Analysis) MVM(16#FFFF,@5babdfcf@,@ccd6cb64@.Util.Block.InterruptComplete.Analysis) [OTU(@ccd6cb64@.Util.Block.InterruptPending.Now) ,FLL(0,@ccd6cb64@.Util.Buffer.Analysis[@5f50ac7e@*66],66) ] ];
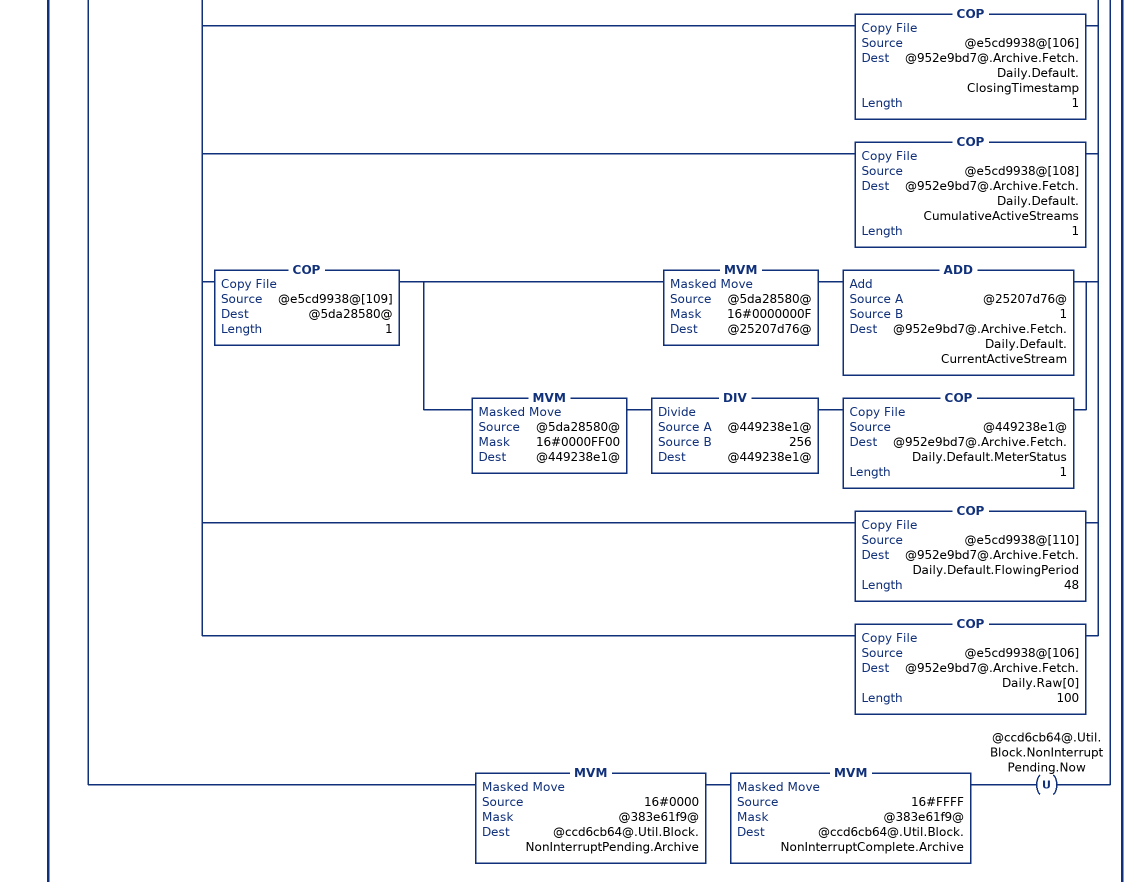
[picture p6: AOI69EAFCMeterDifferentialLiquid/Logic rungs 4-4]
   // Archive Fetch to default and raw UDT's.
   // Get archive alarms.
   // Remove trigger and pending flags.
   4: XIC(@447f2ec8@)CMP(@e5cd9938@[0]=6000+@f89c236e@)[XIC(@952e9bd7@.Archive.Fetch.Hourly.Trigger) [OTU(@952e9bd7@.Archive.Fetch.Hourly.Trigger) ,[[XIC(@e5cd9938@[3].0) OTL(@952e9bd7@.Archive.Fetch.Hourly.Error.ArchiveSelectionInvalid) ,XIO(@e5cd9938@[3].0) OTU(@952e9bd7@.Archive.Fetch.Hourly.Error.ArchiveSelectionInvalid) ] ,[XIC(@e5cd9938@[3].1) OTL(@952e9bd7@.Archive.Fetch.Hourly.Error.AgeOutsideSize) ,XIO(@e5cd9938@[3].1) OTU(@952e9bd7@.Archive.Fetch.Hourly.Error.AgeOutsideSize) ] ,[XIC(@e5cd9938@[3].2) OTL(@952e9bd7@.Archive.Fetch.Hourly.Error.ArchiveNeverWritten) ,XIO(@e5cd9938@[3].2) OTU(@952e9bd7@.Archive.Fetch.Hourly.Error.ArchiveNeverWritten) ] ] ,COP(@e5cd9938@[4],@952e9bd7@.Archive.Fetch.Hourly.Default.ClosingTimestamp,1) ,COP(@e5cd9938@[6],@952e9bd7@.Archive.Fetch.Hourly.Default.CumulativeActiveStreams,1) ,COP(@e5cd9938@[7],@5da28580@,1) [MVM(@5da28580@,16#0000000F,@25207d76@) ADD(@25207d76@,1,@952e9bd7@.Archive.Fetch.Hourly.Default.CurrentActiveStream) ,MVM(@5da28580@,16#0000FF00,@449238e1@) DIV(@449238e1@,256,@449238e1@) COP(@449238e1@,@952e9bd7@.Archive.Fetch.Hourly.Default.MeterStatus,1) ] ,COP(@e5cd9938@[8],@952e9bd7@.Archive.Fetch.Hourly.Default.FlowingPeriod,48) ,COP(@e5cd9938@[4],@952e9bd7@.Archive.Fetch.Hourly.Raw[0],100) ] ,XIC(@952e9bd7@.Archive.Fetch.Daily.Trigger) [OTU(@952e9bd7@.Archive.Fetch.Daily.Trigger) ,[[XIC(@e5cd9938@[105].0) OTL(@952e9bd7@.Archive.Fetch.Daily.Error.ArchiveSelectionInvalid) ,XIO(@e5cd9938@[105].0) OTU(@952e9bd7@.Archive.Fetch.Daily.Error.ArchiveSelectionInvalid) ] ,[XIC(@e5cd9938@[105].1) OTL(@952e9bd7@.Archive.Fetch.Daily.Error.AgeOutsideSize) ,XIO(@e5cd9938@[105].1) OTU(@952e9bd7@.Archive.Fetch.Daily.Error.AgeOutsideSize) ] ,[XIC(@e5cd9938@[105].2) OTL(@952e9bd7@.Archive.Fetch.Daily.Error.ArchiveNeverWritten) ,XIO(@e5cd9938@[105].2) OTU(@952e9bd7@.Archive.Fetch.Daily.Error.ArchiveNeverWritten) ] ] ,COP(@e5cd9938@[106],@952e9bd7@.Archive.Fetch.Daily.Default.ClosingTimestamp,1) ,COP(@e5cd9938@[108],@952e9bd7@.Archive.Fetch.Daily.Default.CumulativeActiveStreams,1) ,COP(@e5cd9938@[109],@5da28580@,1) [MVM(@5da28580@,16#0000000F,@25207d76@) ADD(@25207d76@,1,@952e9bd7@.Archive.Fetch.Daily.Default.CurrentActiveStream) ,MVM(@5da28580@,16#0000FF00,@449238e1@) DIV(@449238e1@,256,@449238e1@) COP(@449238e1@,@952e9bd7@.Archive.Fetch.Daily.Default.MeterStatus,1) ] ,COP(@e5cd9938@[110],@952e9bd7@.Archive.Fetch.Daily.Default.FlowingPeriod,48) ,COP(@e5cd9938@[106],@952e9bd7@.Archive.Fetch.Daily.Raw[0],100) ] ,MVM(16#0000,@383e61f9@,@ccd6cb64@.Util.Block.NonInterruptPending.Archive) MVM(16#FFFF,@383e61f9@,@ccd6cb64@.Util.Block.NonInterruptComplete.Archive) OTU(@ccd6cb64@.Util.Block.NonInterruptPending.Now) ];
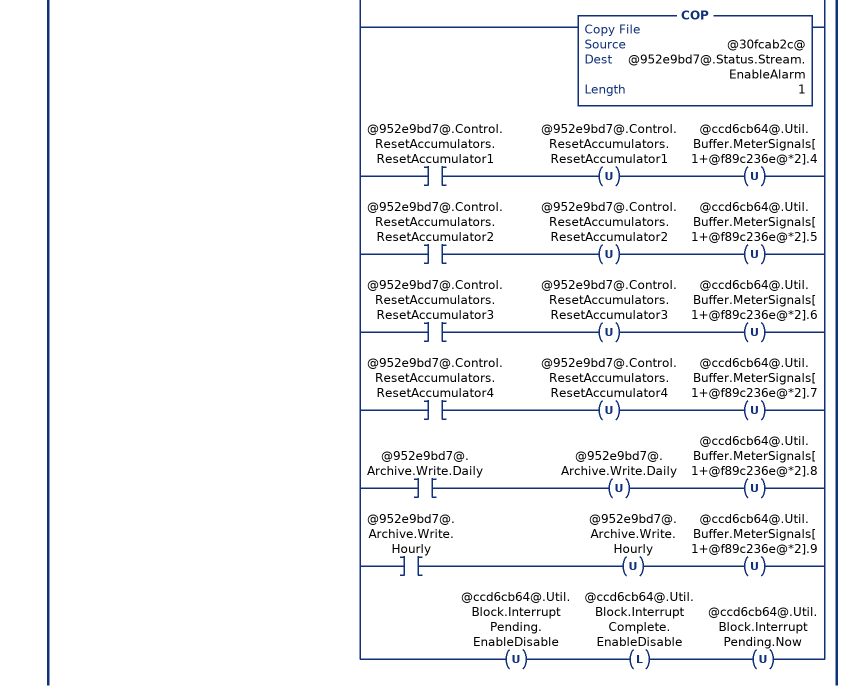
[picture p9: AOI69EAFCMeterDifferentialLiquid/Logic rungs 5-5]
   // Meter status and stream status.
   // Remove trigger and pending flags.
   5: XIC(@447f2ec8@)EQU(@e5cd9938@[0],7000)[[MVM(@e5cd9938@[3],@383e61f9@,@3168918b@) ,[NEQ(@3168918b@,0) OTL(@952e9bd7@.Status.Meter.Enabled) ,EQU(@3168918b@,0) OTU(@952e9bd7@.Status.Meter.Enabled) ] ,OTU(@952e9bd7@.Control.Meter.Enable) MVM(16#0000,@383e61f9@,@ccd6cb64@.Util.Buffer.MeterEnableDisable[1]) ,OTU(@952e9bd7@.Control.Meter.Disable) MVM(16#0000,@383e61f9@,@ccd6cb64@.Util.Buffer.MeterEnableDisable[3]) ] ,[XIC(@952e9bd7@.Control.Stream.EnableSelected) [COP(@e5cd9938@[7+@f89c236e@*3],@952e9bd7@.Status.Stream.Enabled,1) ,COP(@e5cd9938@[8+@f89c236e@*3],@952e9bd7@.Status.Stream.Configured,1) ,OTU(@952e9bd7@.Control.Stream.EnableSelected) OTU(@952e9bd7@.Control.Stream.DisableSelected) ] ,XIC(@952e9bd7@.Control.Stream.DisableSelected) [COP(@e5cd9938@[55+@f89c236e@*3],@952e9bd7@.Status.Stream.Enabled,1) ,COP(@e5cd9938@[56+@f89c236e@*3],@952e9bd7@.Status.Stream.Configured,1) ,OTU(@952e9bd7@.Control.Stream.EnableSelected) OTU(@952e9bd7@.Control.Stream.DisableSelected) ] ] ,[OTU(@952e9bd7@.Control.Stream.SetSelectedToActive) ,COP(@e5cd9938@[103+@f89c236e@*2],@3dde77a8@,1) ,[XIC(@3dde77a8@.8) OTL(@30fcab2c@.0) ,XIO(@3dde77a8@.8) OTU(@30fcab2c@.0) ] ,[XIC(@3dde77a8@.9) OTL(@30fcab2c@.1) ,XIO(@3dde77a8@.9) OTU(@30fcab2c@.1) ] ,[XIC(@3dde77a8@.10) OTL(@30fcab2c@.2) ,XIO(@3dde77a8@.10) OTU(@30fcab2c@.2) ] ,[XIC(@3dde77a8@.11) OTL(@30fcab2c@.3) ,XIO(@3dde77a8@.11) OTU(@30fcab2c@.3) ] ,MVM(@3dde77a8@,16#000F,@19c11729@) ADD(@19c11729@,1,@952e9bd7@.Status.Stream.Active) ,COP(@30fcab2c@,@952e9bd7@.Status.Stream.EnableAlarm,1) ] ,[XIC(@952e9bd7@.Control.ResetAccumulators.ResetAccumulator1) OTU(@952e9bd7@.Control.ResetAccumulators.ResetAccumulator1) OTU(@ccd6cb64@.Util.Buffer.MeterSignals[1+@f89c236e@*2].4) ,XIC(@952e9bd7@.Control.ResetAccumulators.ResetAccumulator2) OTU(@952e9bd7@.Control.ResetAccumulators.ResetAccumulator2) OTU(@ccd6cb64@.Util.Buffer.MeterSignals[1+@f89c236e@*2].5) ,XIC(@952e9bd7@.Control.ResetAccumulators.ResetAccumulator3) OTU(@952e9bd7@.Control.ResetAccumulators.ResetAccumulator3) OTU(@ccd6cb64@.Util.Buffer.MeterSignals[1+@f89c236e@*2].6) ,XIC(@952e9bd7@.Control.ResetAccumulators.ResetAccumulator4) OTU(@952e9bd7@.Control.ResetAccumulators.ResetAccumulator4) OTU(@ccd6cb64@.Util.Buffer.MeterSignals[1+@f89c236e@*2].7) ,XIC(@952e9bd7@.Archive.Write.Daily) OTU(@952e9bd7@.Archive.Write.Daily) OTU(@ccd6cb64@.Util.Buffer.MeterSignals[1+@f89c236e@*2].8) ,XIC(@952e9bd7@.Archive.Write.Hourly) OTU(@952e9bd7@.Archive.Write.Hourly) OTU(@ccd6cb64@.Util.Buffer.MeterSignals[1+@f89c236e@*2].9) ] ,OTU(@ccd6cb64@.Util.Block.InterruptPending.EnableDisable) OTL(@ccd6cb64@.Util.Block.InterruptComplete.EnableDisable) OTU(@ccd6cb64@.Util.Block.InterruptPending.Now) ];
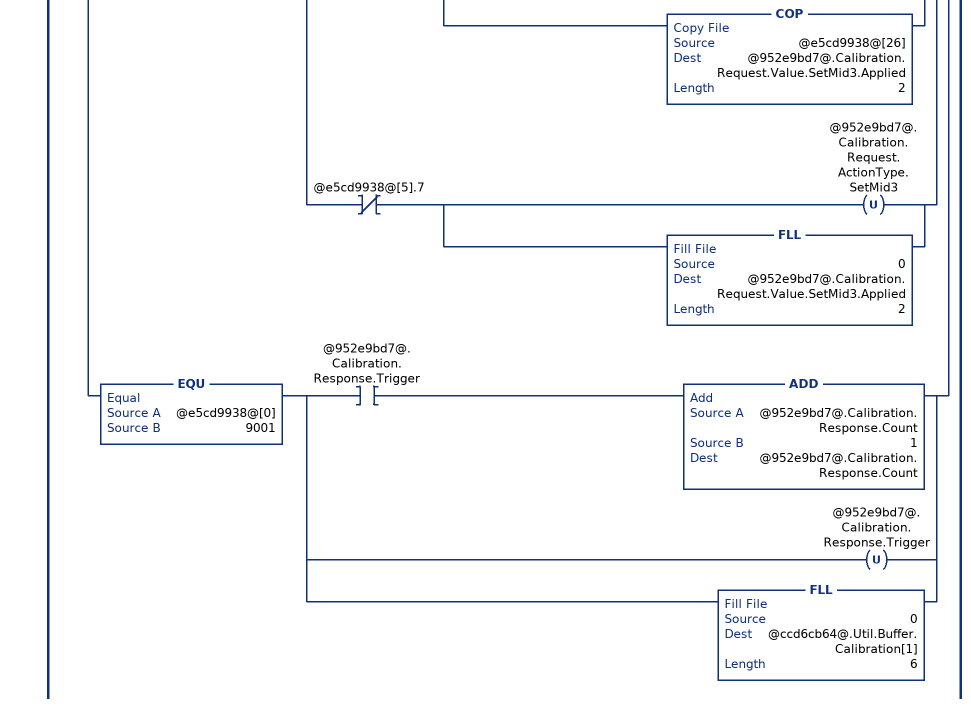
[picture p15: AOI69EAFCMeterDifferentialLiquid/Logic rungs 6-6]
   // Meter transmitter calibration.
   6: XIC(@447f2ec8@)[EQU(@e5cd9938@[0],9000) ,EQU(@e5cd9938@[0],9001) ][MVM(@e5cd9938@[3],16#0F00,@63ef66db@) ,DIV(@63ef66db@,16#100,@63ef66db@) ]EQU(@63ef66db@,@f89c236e@)XIO(@e5cd9938@[3].14)[EQU(@e5cd9938@[0],9000) [XIO(@99473fd2@) ADD(@952e9bd7@.Calibration.Request.Count,1,@952e9bd7@.Calibration.Request.Count) ,OTL(@99473fd2@) [COP(@e5cd9938@[3],@989351bc@,1) ,MVM(@989351bc@,16#000F,@90f69b4d@) ] ,[EQU(@90f69b4d@,0) [OTL(@952e9bd7@.Calibration.Request.ProcessVariable.DifferentialPressure) ,OTU(@952e9bd7@.Calibration.Request.ProcessVariable.Temperature) ,OTU(@952e9bd7@.Calibration.Request.ProcessVariable.Pressure) ,OTU(@952e9bd7@.Calibration.Request.ProcessVariable.Density) ,OTU(@952e9bd7@.Calibration.Request.ProcessVariable.WaterContent) ] ,EQU(@90f69b4d@,1) [OTL(@952e9bd7@.Calibration.Request.ProcessVariable.Temperature) ,OTU(@952e9bd7@.Calibration.Request.ProcessVariable.DifferentialPressure) ,OTU(@952e9bd7@.Calibration.Request.ProcessVariable.Pressure) ,OTU(@952e9bd7@.Calibration.Request.ProcessVariable.Density) ,OTU(@952e9bd7@.Calibration.Request.ProcessVariable.WaterContent) ] ,EQU(@90f69b4d@,2) [OTL(@952e9bd7@.Calibration.Request.ProcessVariable.Pressure) ,OTU(@952e9bd7@.Calibration.Request.ProcessVariable.DifferentialPressure) ,OTU(@952e9bd7@.Calibration.Request.ProcessVariable.Temperature) ,OTU(@952e9bd7@.Calibration.Request.ProcessVariable.Density) ,OTU(@952e9bd7@.Calibration.Request.ProcessVariable.WaterContent) ] ,EQU(@90f69b4d@,3) [OTL(@952e9bd7@.Calibration.Request.ProcessVariable.Density) ,OTU(@952e9bd7@.Calibration.Request.ProcessVariable.DifferentialPressure) ,OTU(@952e9bd7@.Calibration.Request.ProcessVariable.Temperature) ,OTU(@952e9bd7@.Calibration.Request.ProcessVariable.Pressure) ,OTU(@952e9bd7@.Calibration.Request.ProcessVariable.WaterContent) ] ,EQU(@90f69b4d@,4) [OTL(@952e9bd7@.Calibration.Request.ProcessVariable.WaterContent) ,OTU(@952e9bd7@.Calibration.Request.ProcessVariable.DifferentialPressure) ,OTU(@952e9bd7@.Calibration.Request.ProcessVariable.Temperature) ,OTU(@952e9bd7@.Calibration.Request.ProcessVariable.Pressure) ,OTU(@952e9bd7@.Calibration.Request.ProcessVariable.Density) ] ] ,[[XIC(@e5cd9938@[5].2) [OTL(@952e9bd7@.Calibration.Request.ActionType.ZeroShift) ,COP(@e5cd9938@[6],@952e9bd7@.Calibration.Request.Value.ZeroShift.Applied,2) ] ,XIO(@e5cd9938@[5].2) [OTU(@952e9bd7@.Calibration.Request.ActionType.ZeroShift) ,FLL(0,@952e9bd7@.Calibration.Request.Value.ZeroShift.Applied,2) ] ] ,[XIC(@e5cd9938@[5].3) [OTL(@952e9bd7@.Calibration.Request.ActionType.SetZero) ,COP(@e5cd9938@[10],@952e9bd7@.Calibration.Request.Value.SetZero.Applied,2) ] ,XIO(@e5cd9938@[5].3) [OTU(@952e9bd7@.Calibration.Request.ActionType.SetZero) ,FLL(0,@952e9bd7@.Calibration.Request.Value.SetZero.Applied,2) ] ] ,[XIC(@e5cd9938@[5].4) [OTL(@952e9bd7@.Calibration.Request.ActionType.SetSpan) ,COP(@e5cd9938@[14],@952e9bd7@.Calibration.Request.Value.SetSpan.Applied,2) ] ,XIO(@e5cd9938@[5].4) [OTU(@952e9bd7@.Calibration.Request.ActionType.SetSpan) ,FLL(0,@952e9bd7@.Calibration.Request.Value.SetSpan.Applied,2) ] ] ,[XIC(@e5cd9938@[5].5) [OTL(@952e9bd7@.Calibration.Request.ActionType.SetMid1) ,COP(@e5cd9938@[18],@952e9bd7@.Calibration.Request.Value.SetMid1.Applied,2) ] ,XIO(@e5cd9938@[5].5) [OTU(@952e9bd7@.Calibration.Request.ActionType.SetMid1) ,FLL(0,@952e9bd7@.Calibration.Request.Value.SetMid1.Applied,2) ] ] ,[XIC(@e5cd9938@[5].6) [OTL(@952e9bd7@.Calibration.Request.ActionType.SetMid2) ,COP(@e5cd9938@[22],@952e9bd7@.Calibration.Request.Value.SetMid2.Applied,2) ] ,XIO(@e5cd9938@[5].6) [OTU(@952e9bd7@.Calibration.Request.ActionType.SetMid2) ,FLL(0,@952e9bd7@.Calibration.Request.Value.SetMid2.Applied,2) ] ] ,[XIC(@e5cd9938@[5].7) [OTL(@952e9bd7@.Calibration.Request.ActionType.SetMid3) ,COP(@e5cd9938@[26],@952e9bd7@.Calibration.Request.Value.SetMid3.Applied,2) ] ,XIO(@e5cd9938@[5].7) [OTU(@952e9bd7@.Calibration.Request.ActionType.SetMid3) ,FLL(0,@952e9bd7@.Calibration.Request.Value.SetMid3.Applied,2) ] ] ] ] ,EQU(@e5cd9938@[0],9001) [XIC(@952e9bd7@.Calibration.Response.Trigger) ADD(@952e9bd7@.Calibration.Response.Count,1,@952e9bd7@.Calibration.Response.Count) ,OTU(@952e9bd7@.Calibration.Response.Trigger) ,FLL(0,@ccd6cb64@.Util.Buffer.Calibration[1],6) ] ];
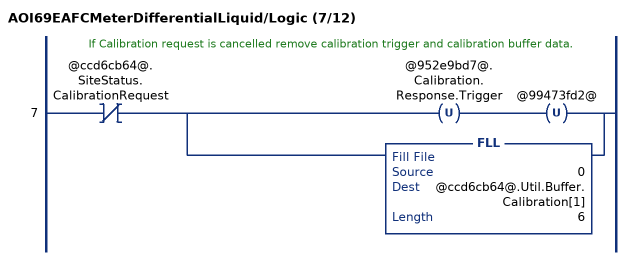
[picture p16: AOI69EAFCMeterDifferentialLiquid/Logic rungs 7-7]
   // If Calibration request is cancelled remove calibration trigger and calibration buffer data.
   7: XIO(@ccd6cb64@.SiteStatus.CalibrationRequest)[OTU(@952e9bd7@.Calibration.Response.Trigger) OTU(@99473fd2@) ,FLL(0,@ccd6cb64@.Util.Buffer.Calibration[1],6) ];
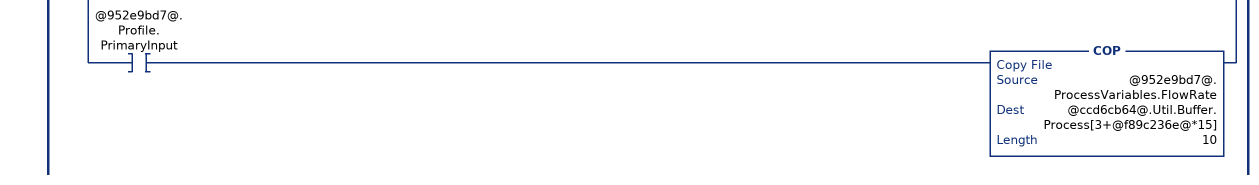
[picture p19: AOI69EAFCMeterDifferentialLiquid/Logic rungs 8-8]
   // Process variables and process alarms to send to module.
   8: XIC(@73ebb0c9@)[ADD(16#A000,@911e6e5e@,@633827b3@) COP(@633827b3@,@ccd6cb64@.Util.Buffer.Process[@f89c236e@*15],1) ,[XIO(@952e9bd7@.Profile.PrimaryInput) XIC(@952e9bd7@.Alarm.Control.DifferentialPressure.SetAutoClearStaleData) OTU(@952e9bd7@.Alarm.Control.DifferentialPressure.StaleData) ,XIC(@952e9bd7@.Profile.PrimaryInput) XIC(@952e9bd7@.Alarm.Control.FlowRate.SetAutoClearStaleData) OTU(@952e9bd7@.Alarm.Control.FlowRate.StaleData) ,XIO(@952e9bd7@.Profile.PrimaryInput) COP(@952e9bd7@.Alarm.Control.DifferentialPressure,@ccd6cb64@.Util.Buffer.Process[1+@f89c236e@*15],1) OTL(@952e9bd7@.Alarm.Control.DifferentialPressure.StaleData) ,XIC(@952e9bd7@.Profile.PrimaryInput) COP(@952e9bd7@.Alarm.Control.FlowRate,@ccd6cb64@.Util.Buffer.Process[1+@f89c236e@*15],1) OTL(@952e9bd7@.Alarm.Control.FlowRate.StaleData) ] ,[XIC(@952e9bd7@.Alarm.Control.Temperature.SetAutoClearStaleData) OTU(@952e9bd7@.Alarm.Control.Temperature.StaleData) ,COP(@952e9bd7@.Alarm.Control.Temperature,@7b7177f4@,1) MUL(@7b7177f4@,16,@db56644a@) MVM(@db56644a@,16#00F0,@ccd6cb64@.Util.Buffer.Process[1+@f89c236e@*15]) OTL(@952e9bd7@.Alarm.Control.Temperature.StaleData) ] ,[XIC(@952e9bd7@.Alarm.Control.Pressure.SetAutoClearStaleData) OTU(@952e9bd7@.Alarm.Control.Pressure.StaleData) ,COP(@952e9bd7@.Alarm.Control.Pressure,@7b7177f4@,1) MUL(@7b7177f4@,256,@db56644a@) MVM(@db56644a@,16#0F00,@ccd6cb64@.Util.Buffer.Process[1+@f89c236e@*15]) MVM(@ccd6cb64@.Util.Buffer.Process[1+@f89c236e@*15],16#0FFF,@d4f958e5@) OTL(@952e9bd7@.Alarm.Control.Pressure.StaleData) ] ,[XIC(@952e9bd7@.Alarm.Control.Density.SetAutoClearStaleData) OTU(@952e9bd7@.Alarm.Control.Density.SetAutoClearStaleData) ,COP(@952e9bd7@.Alarm.Control.Density,@7b7177f4@,1) MUL(@7b7177f4@,4096,@db56644a@) MVM(@db56644a@,16#F000,@d4f958e5@) COP(@d4f958e5@,@ccd6cb64@.Util.Buffer.Process[1+@f89c236e@*15],1) OTL(@952e9bd7@.Alarm.Control.Density.SetAutoClearStaleData) ] ,[XIC(@952e9bd7@.Alarm.Control.WaterPercent.SetAutoClearStaleData) OTU(@952e9bd7@.Alarm.Control.WaterPercent.SetAutoClearStaleData) ,COP(@952e9bd7@.Alarm.Control.WaterPercent,@ccd6cb64@.Util.Buffer.Process[2+@f89c236e@*15],2) OTL(@952e9bd7@.Alarm.Control.WaterPercent.SetAutoClearStaleData) ] ,COP(@952e9bd7@.Alarm.Control.WaterPercent,@7b7177f4@,1) MUL(@7b7177f4@,16,@db56644a@) MVM(@db56644a@,16#00F0,@ccd6cb64@.Util.Buffer.Process[2+@f89c236e@*15]) ,XIO(@952e9bd7@.Profile.PrimaryInput) [COP(@952e9bd7@.ProcessVariables.DifferentialPressure,@ccd6cb64@.Util.Buffer.Process[3+@f89c236e@*15],2) ,COP(@952e9bd7@.ProcessVariables.Temperature,@ccd6cb64@.Util.Buffer.Process[3+2+@f89c236e@*15],8) ] ,XIC(@952e9bd7@.Profile.PrimaryInput) COP(@952e9bd7@.ProcessVariables.FlowRate,@ccd6cb64@.Util.Buffer.Process[3+@f89c236e@*15],10) ];
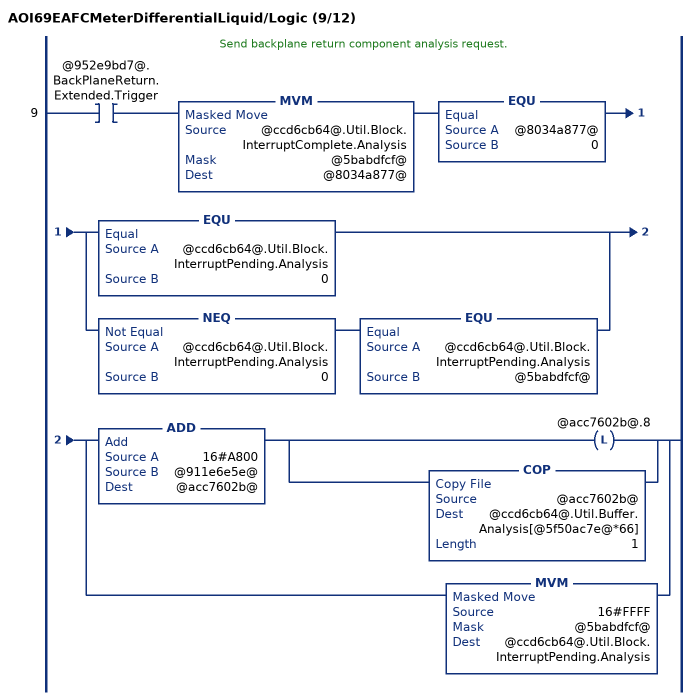
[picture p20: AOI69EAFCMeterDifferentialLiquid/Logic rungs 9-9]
   // Send backplane return component analysis request.
   9: XIC(@952e9bd7@.BackPlaneReturn.Extended.Trigger)MVM(@ccd6cb64@.Util.Block.InterruptComplete.Analysis,@5babdfcf@,@8034a877@)EQU(@8034a877@,0)[EQU(@ccd6cb64@.Util.Block.InterruptPending.Analysis,0) ,NEQ(@ccd6cb64@.Util.Block.InterruptPending.Analysis,0) EQU(@ccd6cb64@.Util.Block.InterruptPending.Analysis,@5babdfcf@) ][ADD(16#A800,@911e6e5e@,@acc7602b@) [OTL(@acc7602b@.8) ,COP(@acc7602b@,@ccd6cb64@.Util.Buffer.Analysis[@5f50ac7e@*66],1) ] ,MVM(16#FFFF,@5babdfcf@,@ccd6cb64@.Util.Block.InterruptPending.Analysis) ];
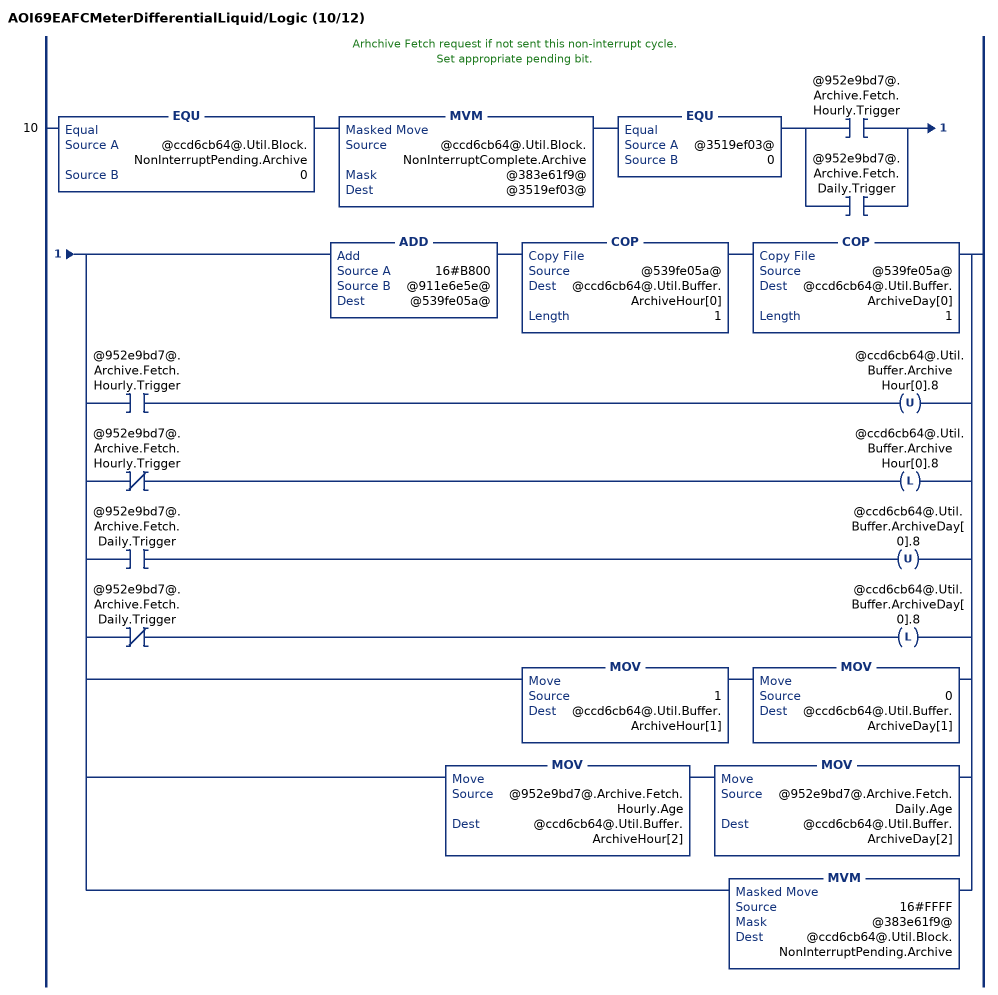
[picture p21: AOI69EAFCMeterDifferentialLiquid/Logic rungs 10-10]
   // Arhchive Fetch request if not sent this non-interrupt cycle.
   // Set appropriate pending bit.
   10: EQU(@ccd6cb64@.Util.Block.NonInterruptPending.Archive,0)MVM(@ccd6cb64@.Util.Block.NonInterruptComplete.Archive,@383e61f9@,@3519ef03@)EQU(@3519ef03@,0)[XIC(@952e9bd7@.Archive.Fetch.Hourly.Trigger) ,XIC(@952e9bd7@.Archive.Fetch.Daily.Trigger) ][ADD(16#B800,@911e6e5e@,@539fe05a@) COP(@539fe05a@,@ccd6cb64@.Util.Buffer.ArchiveHour[0],1) COP(@539fe05a@,@ccd6cb64@.Util.Buffer.ArchiveDay[0],1) ,[XIC(@952e9bd7@.Archive.Fetch.Hourly.Trigger) OTU(@ccd6cb64@.Util.Buffer.ArchiveHour[0].8) ,XIO(@952e9bd7@.Archive.Fetch.Hourly.Trigger) OTL(@ccd6cb64@.Util.Buffer.ArchiveHour[0].8) ] ,[XIC(@952e9bd7@.Archive.Fetch.Daily.Trigger) OTU(@ccd6cb64@.Util.Buffer.ArchiveDay[0].8) ,XIO(@952e9bd7@.Archive.Fetch.Daily.Trigger) OTL(@ccd6cb64@.Util.Buffer.ArchiveDay[0].8) ] ,MOV(1,@ccd6cb64@.Util.Buffer.ArchiveHour[1]) MOV(0,@ccd6cb64@.Util.Buffer.ArchiveDay[1]) ,MOV(@952e9bd7@.Archive.Fetch.Hourly.Age,@ccd6cb64@.Util.Buffer.ArchiveHour[2]) MOV(@952e9bd7@.Archive.Fetch.Daily.Age,@ccd6cb64@.Util.Buffer.ArchiveDay[2]) ,MVM(16#FFFF,@383e61f9@,@ccd6cb64@.Util.Block.NonInterruptPending.Archive) ];
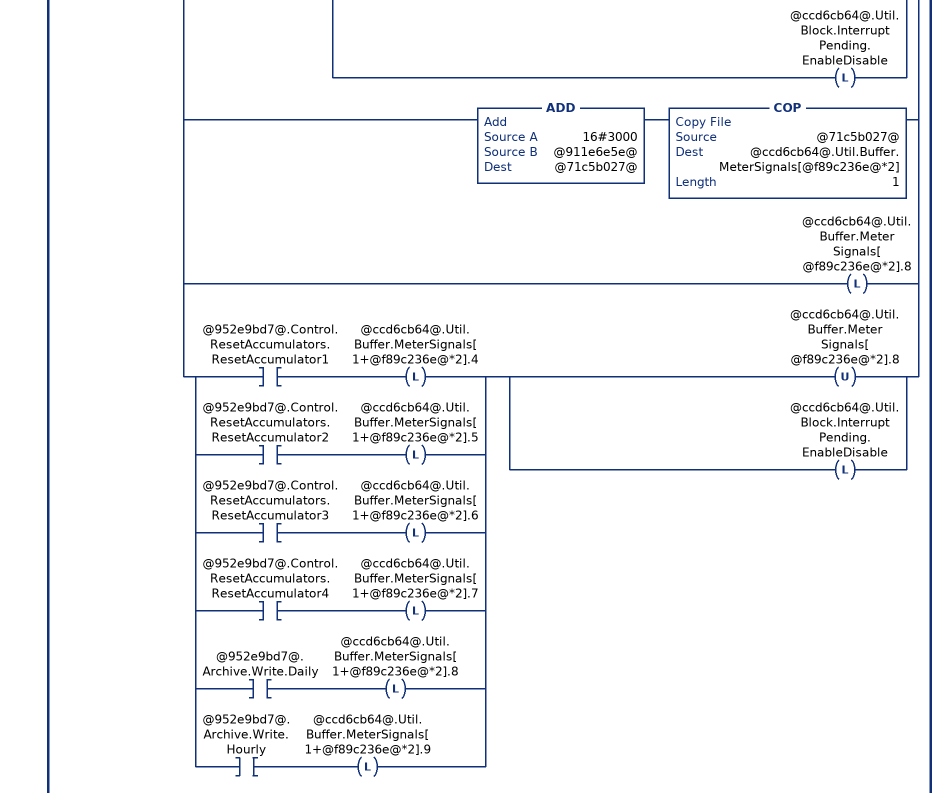
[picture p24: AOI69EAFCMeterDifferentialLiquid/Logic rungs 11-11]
   // Meter Enable.
   // Meter Disable.
   // Stream Select.
   // Stream Enable.
   // Stream Disable.
   // Set pending bit if not set this interrupt cycle.
   11: XIO(@ccd6cb64@.Util.Block.InterruptComplete.EnableDisable)[LIM(1,@952e9bd7@.Control.Stream.Selected,16) CPT(@03387e66@,2**(@952e9bd7@.Control.Stream.Selected-1)) ,[XIC(@952e9bd7@.Control.Meter.Enable) MVM(16#FFFF,@383e61f9@,@ccd6cb64@.Util.Buffer.MeterEnableDisable[1]) MVM(16#0000,@383e61f9@,@ccd6cb64@.Util.Buffer.MeterEnableDisable[3]) ,XIC(@952e9bd7@.Control.Meter.Disable) MVM(16#FFFF,@383e61f9@,@ccd6cb64@.Util.Buffer.MeterEnableDisable[3]) MVM(16#0000,@383e61f9@,@ccd6cb64@.Util.Buffer.MeterEnableDisable[1]) ] OTL(@ccd6cb64@.Util.Block.InterruptPending.EnableDisable) ,[ADD(16#CC00,@911e6e5e@,@7504797f@) COP(@7504797f@,@ccd6cb64@.Util.Buffer.StreamEnable[@f89c236e@*3],1) ,XIO(@952e9bd7@.Control.Stream.EnableSelected) OTL(@ccd6cb64@.Util.Buffer.StreamEnable[@f89c236e@*3].8) ,XIC(@952e9bd7@.Control.Stream.EnableSelected) [OTU(@ccd6cb64@.Util.Buffer.StreamEnable[@f89c236e@*3].8) ,COP(@03387e66@,@ccd6cb64@.Util.Buffer.StreamEnable[1+@f89c236e@*3],1) ,OTL(@ccd6cb64@.Util.Block.InterruptPending.EnableDisable) ] ] ,[ADD(16#C800,@911e6e5e@,@5d1d8c11@) COP(@5d1d8c11@,@ccd6cb64@.Util.Buffer.StreamDisable[@f89c236e@*3],1) ,XIO(@952e9bd7@.Control.Stream.DisableSelected) OTL(@ccd6cb64@.Util.Buffer.StreamDisable[@f89c236e@*3].8) ,XIC(@952e9bd7@.Control.Stream.DisableSelected) [OTU(@ccd6cb64@.Util.Buffer.StreamDisable[@f89c236e@*3].8) ,COP(@03387e66@,@ccd6cb64@.Util.Buffer.StreamDisable[1+@f89c236e@*3],1) ,OTL(@ccd6cb64@.Util.Block.InterruptPending.EnableDisable) ] ] ,[ADD(16#3C00,@911e6e5e@,@beac2dc2@) COP(@beac2dc2@,@ccd6cb64@.Util.Buffer.StreamSelect[@f89c236e@*2],1) ,XIO(@952e9bd7@.Control.Stream.SetSelectedToActive) OTL(@ccd6cb64@.Util.Buffer.StreamSelect[@f89c236e@*2].8) ,XIC(@952e9bd7@.Control.Stream.SetSelectedToActive) [OTU(@ccd6cb64@.Util.Buffer.StreamSelect[@f89c236e@*2].8) ,MOV(@952e9bd7@.Control.Stream.Selected,@ccd6cb64@.Util.Buffer.StreamSelect[1+@f89c236e@*2]) ,OTL(@ccd6cb64@.Util.Block.InterruptPending.EnableDisable) ] ] ,[ADD(16#3000,@911e6e5e@,@71c5b027@) COP(@71c5b027@,@ccd6cb64@.Util.Buffer.MeterSignals[@f89c236e@*2],1) ,OTL(@ccd6cb64@.Util.Buffer.MeterSignals[@f89c236e@*2].8) ,[XIC(@952e9bd7@.Control.ResetAccumulators.ResetAccumulator1) OTL(@ccd6cb64@.Util.Buffer.MeterSignals[1+@f89c236e@*2].4) ,XIC(@952e9bd7@.Control.ResetAccumulators.ResetAccumulator2) OTL(@ccd6cb64@.Util.Buffer.MeterSignals[1+@f89c236e@*2].5) ,XIC(@952e9bd7@.Control.ResetAccumulators.ResetAccumulator3) OTL(@ccd6cb64@.Util.Buffer.MeterSignals[1+@f89c236e@*2].6) ,XIC(@952e9bd7@.Control.ResetAccumulators.ResetAccumulator4) OTL(@ccd6cb64@.Util.Buffer.MeterSignals[1+@f89c236e@*2].7) ,XIC(@952e9bd7@.Archive.Write.Daily) OTL(@ccd6cb64@.Util.Buffer.MeterSignals[1+@f89c236e@*2].8) ,XIC(@952e9bd7@.Archive.Write.Hourly) OTL(@ccd6cb64@.Util.Buffer.MeterSignals[1+@f89c236e@*2].9) ] [OTU(@ccd6cb64@.Util.Buffer.MeterSignals[@f89c236e@*2].8) ,OTL(@ccd6cb64@.Util.Block.InterruptPending.EnableDisable) ] ] ];
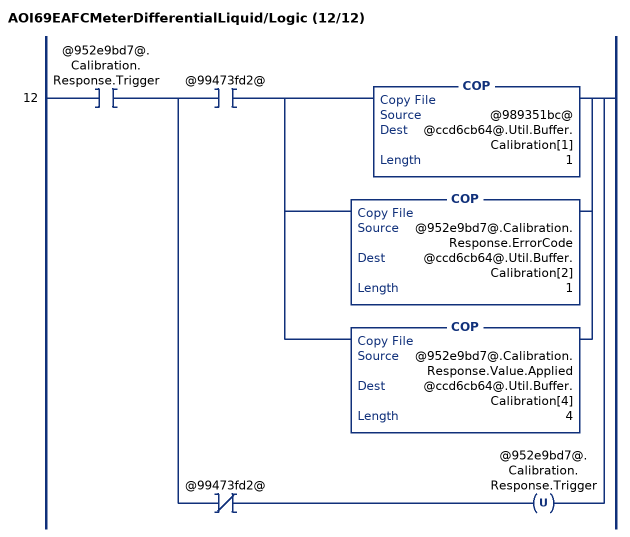
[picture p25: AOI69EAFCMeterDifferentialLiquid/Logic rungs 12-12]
   12: XIC(@952e9bd7@.Calibration.Response.Trigger)[XIC(@99473fd2@) [COP(@989351bc@,@ccd6cb64@.Util.Buffer.Calibration[1],1) ,COP(@952e9bd7@.Calibration.Response.ErrorCode,@ccd6cb64@.Util.Buffer.Calibration[2],1) ,COP(@952e9bd7@.Calibration.Response.Value.Applied,@ccd6cb64@.Util.Buffer.Calibration[4],4) ] ,XIO(@99473fd2@) OTU(@952e9bd7@.Calibration.Response.Trigger) ];
END_ROUTINE

ROUTINE Prescan   (* ladder *)
// Prescan
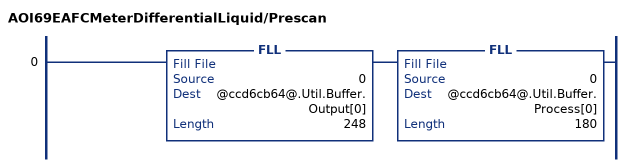
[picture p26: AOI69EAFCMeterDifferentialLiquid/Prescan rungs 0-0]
   0: FLL(0,@ccd6cb64@.Util.Buffer.Output[0],248)FLL(0,@ccd6cb64@.Util.Buffer.Process[0],180);
END_ROUTINE
END_ADD_ON_INSTRUCTION

VAR_GLOBAL   (* controller tags *)
   Local:1:I : AB:1756_MODULE_INT_496Bytes:I:0;
   AFC : AFCEModuleDef;
   AFCMeter02DifferentialLiquid : AFCEMeterDifferentialLiquid;
   AOI69EAFCMeter02DifferentialLiquid : AOI69EAFCMeterDifferentialLiquid;
END_VAR

PROGRAM MainProgram

ROUTINE MainRoutine   (* ladder *)
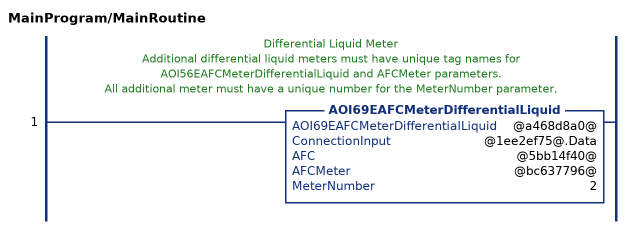
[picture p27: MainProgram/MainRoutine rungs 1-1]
   // Differential Liquid Meter
   // Additional differential liquid meters must have unique tag names for AOI56EAFCMeterDifferentialLiquid and AFCMeter parameters.
   // All additional meter must have a unique number for the MeterNumber parameter.
   1: AOI69EAFCMeterDifferentialLiquid(@a468d8a0@,@1ee2ef75@.Data,@5bb14f40@,@bc637796@,2);
END_ROUTINE
END_PROGRAM
